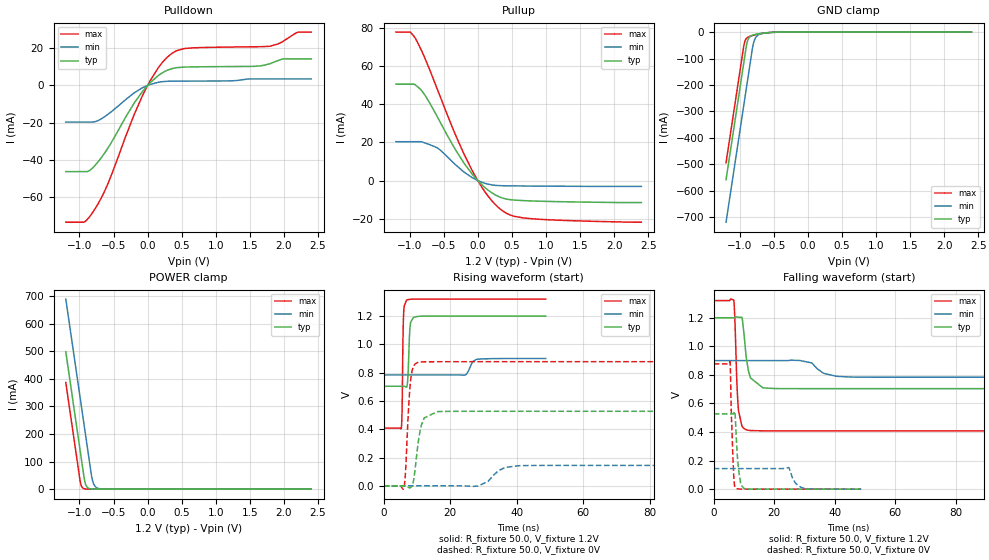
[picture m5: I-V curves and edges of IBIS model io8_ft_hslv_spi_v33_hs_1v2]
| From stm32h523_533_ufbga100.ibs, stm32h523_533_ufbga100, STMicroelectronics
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[Model]   io8_ft_hslv_spi_v33_hs_1v2
Model_type I/O
Polarity   Non-Inverting
Enable   Active-Low
| CAP_THRESHOLD on pad IOFT is "UDTCAPC" :
| Rising=20.0% of vddiom   Falling=80.0% of vddiom
| C_comp min and max val. don't necessarily correlate with the min and max pvt
| but are the smallest and greatest pad capacitance found.
| var   typ   min   max
C_comp   3.39570pF  3.37235pF  3.42695pF
|C_comp_pullup   2.09350pF  2.00500pF  1.90825pF
|C_comp_pulldown   1.30220pF  1.36735pF  1.51870pF
Vinl = 270.0mV
Vinh = 924.0mV
Vmeas = 600.0mV   | Reference voltage for timing measurements
Cref  = 50.0pF   | Timing specification test load capacitance value
Rref  = 100.0MOhm   | Timing specification test load resistance value
Vref  = 600.0mV   | Timing specification test load voltage
[Model Spec]
| TIME_THRESHOLD on pin ZIV33M is "CMOS" :
| Rising=40.0% of vddiom   Falling=60.0% of vddiom
Vinl 437.80000mV 335.80000mV 479.80000mV
Vinh 728.20000mV 529.20000mV 807.20000mV
| variable   typ   min   max
[Temperature Range] 25.0 125.0 -40.0
| variable   typ   min   max
[Voltage Range] 1.2V 900.0mV 1.32V
| variable   typ   min   max
[POWER Clamp Reference] 1.2V 900.0mV 1.32V
| variable   typ   min   max
[GND Clamp Reference] 0V 0V 0V
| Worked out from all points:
|   slope of the pulldown table from 0 to 0.18 V, typ, clamps not added: 30.6 ohm
|   slope of the pullup table from 0 to 0.18 V, typ, clamps not added: 31.2 ohm
|   GND clamp passes 1 mA (typ) near -0.52 V on its own axis
|   POWER clamp passes 1 mA (typ) near -0.84 V on its own axis
|   rising waveform, R_fixture 50.0, V_fixture 1.2V: 20-80 % time 511ps typ, 1.44ns min, 316ps max; typ from 0.704 V to 1.2 V
|   falling waveform, R_fixture 50.0, V_fixture 1.2V: 20-80 % time 1.89ns typ, 4.41ns min, 969ps max; typ from 1.2 V to 0.704 V
|   rising waveform, R_fixture 50.0, V_fixture 0V: 20-80 % time 1.88ns typ, 4.12ns min, 1.19ns max; typ from 0 V to 0.527 V
|   falling waveform, R_fixture 50.0, V_fixture 0V: 20-80 % time 1.12ns typ, 2.26ns min, 794ps max; typ from 0.527 V to 0 V
[POWER Clamp]
-1.2V     497.8mA    689.2mA    386.5mA
-990mV    140.8mA    332.2mA    29.53mA
-980mV    123.8mA    315.2mA    17.95mA
-960mV    89.81mA    281.2mA    6.634mA
-930mV    38.81mA    230.2mA    1.49mA
-900mV    12.07mA    179.2mA    334.8uA
-870mV    3.756mA    128.2mA    75.22uA
-820mV    536.4uA    44.98mA    6.246uA
-790mV    166.9uA    18.76mA    1.403uA
-750mV    35.18uA    5.846mA    191.8nA
-590mV    70.08nA    55uA       163.4pA
2.4V      0A         0A         0A
[GND Clamp]
-1.2V     -558.2mA   -719mA     -494.1mA
-940mV    -116.2mA   -277mA     -52.06mA
-930mV    -99.19mA   -260mA     -39.94mA
-900mV    -49.1mA    -209mA     -23.76mA
-880mV    -30.14mA   -175mA     -19.6mA
-850mV    -17.82mA   -124mA     -16.09mA
-810mV    -11.73mA   -56.78mA   -12.91mA
-780mV    -9.444mA   -28.21mA   -10.92mA
-740mV    -7.291mA   -13.16mA   -8.574mA
-640mV    -3.573mA   -4.171mA   -3.954mA
-380mV    -61.75uA   -230.3uA   -20.32uA
2.4V      3.863nA    718.6nA    150.6pA
| variable   typ   min   max
[Pullup Reference] 1.2V 900.0mV 1.32V
| variable   typ   min   max
[Pulldown Reference] 0V 0V 0V
[Pullup]
-1.2V     50.54mA    20.37mA    77.87mA
-990mV    50.54mA    20.37mA    77.87mA
-920mV    50.27mA    20.37mA    74.87mA
-790mV    45.58mA    19.94mA    65.42mA
-590mV    33.26mA    17.06mA    47.66mA
-330mV    16.36mA    8.406mA    24.24mA
-80mV     3.305mA    1.499mA    5.124mA
130mV     -4.4mA     -1.69mA    -7.128mA
340mV     -8.864mA   -2.692mA   -15.22mA
540mV     -10.25mA   -2.811mA   -18.8mA
760mV     -10.66mA   -2.884mA   -19.93mA
2.4V      -11.55mA   -3.057mA   -21.84mA
[Pulldown]
-1.2V     -46.17mA   -19.62mA   -73.27mA
-930mV    -46.17mA   -19.62mA   -73.18mA
-770mV    -42.8mA    -19.41mA   -66.04mA
-570mV    -32.88mA   -15.18mA   -51.58mA
-80mV     -3.488mA   -1.363mA   -5.887mA
160mV     5.368mA    1.686mA    9.621mA
340mV     8.782mA    2.251mA    16.66mA
540mV     9.805mA    2.305mA    19.74mA
1.79V     11.53mA    3.428mA    20.94mA
1.98V     14.11mA    3.428mA    23.43mA
2.2V      14.2mA     3.428mA    28.44mA
2.4V      14.2mA     3.428mA    28.54mA
[Ramp]
dV/dt_r 315.98501mV/1.8792ns 86.4834mV/3.79242ns 526.35113mV/1.18538ns
dV/dt_f 297.80506mV/1.83382ns 69.9241mV/4.12121ns 547.13926mV/967.39083ps
R_load = 50.0
| Removed startup time: 0s 0s 0s  .
| Removed end time: 48.75ns.
[Rising Waveform]
R_fixture   = 50.0
V_fixture   = 1.2V
V_fixture_min = 900.0mV
V_fixture_max = 1.32V
0s        703.7mV    783.5mV    408.1mV
5.3ns     703.8mV    783.5mV    406.3mV
5.55ns    703.8mV    783.5mV    544.6mV
5.8ns     703.8mV    783.5mV    1.022V
6ns       703.9mV    783.5mV    1.212V
6.85ns    696.6mV    783.5mV    1.311V
7.25ns    755.4mV    783.5mV    1.315V
8ns       1.137V     783.5mV    1.318V
8.95ns    1.19V      783.5mV    1.32V
48.75ns   1.2V       899.9mV    1.32V
| Removed startup time: 0s 0s 0s  .
| Removed end time: 198.75ns.
[Falling Waveform]
R_fixture   = 50.0
V_fixture   = 1.2V
V_fixture_min = 900.0mV
V_fixture_max = 1.32V
0s        1.2V       900mV      1.32V
6.6ns     1.2V       900mV      1.324V
7ns       1.203V     900mV      1.173V
7.7ns     1.205V     900mV      718.4mV
8.2ns     1.203V     900mV      547.5mV
9.4ns     1.196V     900mV      438.6mV
11.45ns   829.3mV    900mV      412.2mV
20.3ns    704.2mV    900mV      408.1mV
44.65ns   703.7mV    785.3mV    408.1mV
198.8ns   703.7mV    783.5mV    408.1mV
| Removed startup time: 0s 0s 0s  .
| Removed end time: 198.7ns.
[Rising Waveform]
R_fixture   = 50.0
V_fixture   = 0V
V_fixture_min = 0V
V_fixture_max = 0V
0s        207.9nV    698.8nV    140.7nV
6.1ns     -14.92uV   704.7nV    -12.97mV
8.2ns     -10.31mV   694.5nV    762.1mV
9.1ns     53.06mV    685nV      849.1mV
10.7ns    354.7mV    657.4nV    873.8mV
12.2ns    479.8mV    610.6nV    876.4mV
16.2ns    524.7mV    150.1nV    877.1mV
28.4ns    526.6mV    -1.824mV   877.2mV
40.6ns    526.6mV    141.9mV    877.2mV
198.7ns   526.6mV    144.1mV    877.3mV
| Removed startup time: 0s 0s 0s  .
| Removed end time: 48.75ns.
[Falling Waveform]
R_fixture   = 50.0
V_fixture   = 0V
V_fixture_min = 0V
V_fixture_max = 0V
0s        526.6mV    144.2mV    877.3mV
5.4ns     526.7mV    144.2mV    889.5mV
5.8ns     526.7mV    144.2mV    532.8mV
6.4ns     526.5mV    144.2mV    186.7mV
7.15ns    492.6mV    144.2mV    8.41mV
8.2ns     137.5mV    144.2mV    1.404mV
9.95ns    4.992mV    144.2mV    266uV
24.65ns   3.586uV    151.5mV    679.5nV
29.9ns    1.142uV    5.961mV    176nV
48.75ns   62.34nV    18.57uV    29.76nV
